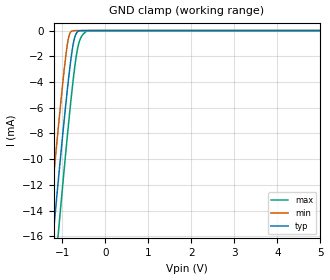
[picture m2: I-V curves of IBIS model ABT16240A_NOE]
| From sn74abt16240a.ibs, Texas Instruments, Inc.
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[Model]   ABT16240A_NOE
Model_type  Input
Vinl = 0.8
Vinh = 2.0
| variable   typ   min   max
C_comp   1.82pF   1.41pF   2.89pF
[Temperature Range]   40   -40   100
| Ambient temperature   25   -40   85
[Voltage range]   5   4.5   5.5
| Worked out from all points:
|   GND clamp passes 1 mA (typ) near -0.74 V on its own axis
[GND Clamp]
| ABT16240A_NOE
|   Voltage   I(typ)   I(min)   I(max)
-5V       -186.6mA   -169.1mA   -195.9mA
-1.345V   -21.02mA   -16.72mA   -25.9mA
-1.3V     -19.33mA   -15.07mA   -23.89mA
-1.19V    -15.28mA   -11.09mA   -19.59mA
-1.075V   -11.16mA   -7.058mA   -15.26mA
-885mV    -4.787mA   -1.222mA   -8.405mA
-830mV    -3.145mA   -304.3uA   -6.541mA
-775mV    -1.717mA   -44.94uA   -4.777mA
-700mV    -444.6uA   -2.089uA   -2.653mA
-615mV    -35.78uA   -37.44nA   -1.014mA
-410mV    -25.36nA   -45.73pA   -20.98uA
5V        88.45pA    93.15pA    937.4pA
